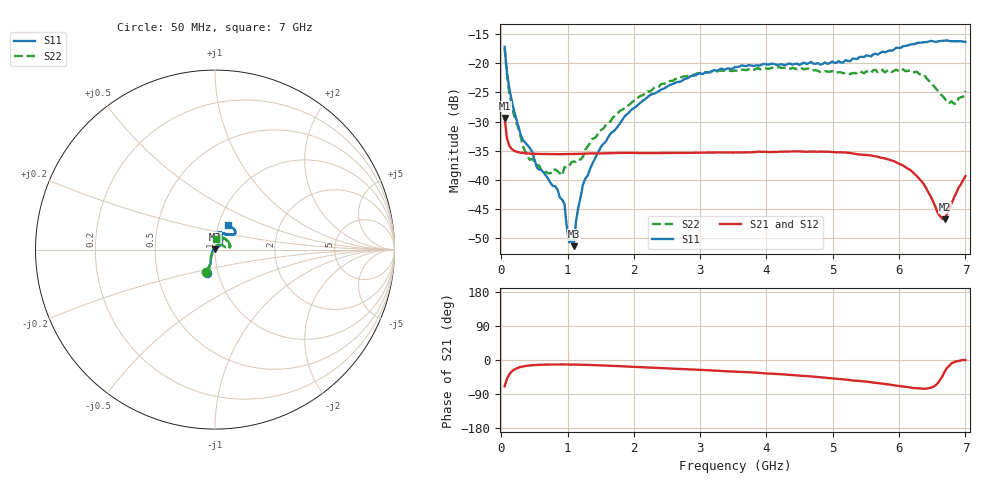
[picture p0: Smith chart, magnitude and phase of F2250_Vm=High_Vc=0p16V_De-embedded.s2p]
! Integrated Device Technology
! Corporate Headquarters
! 6024 Silver Creek Valley Road
! San Jose, CA 95138  USA
! Phone:  1-408-284-8200
! Toll Free:  1-800-223-1366
! Webpage:  http://www.idt.com/
! Timing and RF Division
! 515 Groton Road, Suite 102
! Westford, MA 01886-6024
! Device:  F2250
! Description: Voltage Variable RF Attenuator
! Frequency:  50.0 -  6000.00 MHz
! Package:  3x3 mm Thin QFN Plastic Package: 16 pin
! Ports:  2 RF, 3 DC
!  Pin  1  = GND
!  Pin  2  = NC
!  Pin  3  = RF1  = Port 1
!  Pin  4  = NC
!  Pin  5  = GND
!  Pin  6  = GND
!  Pin  7  = GND
!  Pin  8  = GND
!  Pin  9  = NC
!  Pin 10  = RF2  = Port 2
!  Pin 11  = NC
!  Pin 12  = GND
!  Pin 13  = GND
!  Pin 14  = VCNTRL
!  Pin 15  = VDD
!  Pin 16  = VMODE
! Vcntrl:  0.160 Volts
! Vmode:  +3.300 Volts
! Vdd:  +3.30  Volts
! Current:  1.243 mA
! Data:  The device was measured on a the F2250 evaluation board which has
!  individual transmission lines to the RF pins.  Data was collected
!  using a calibrated network analyzer.  The evaluation board was
!  de-embedded using a TRL calibration technique.
!  The reference plane is the edge of the package pin.
! Misc:  SN 10
!  Action Tracker AT0258
! Date Measured:  2014-11-26
! Date:  2015-10-15  MJV
! Note:
!  Integrated Device Technology supplies this data as a sample of measured
!  data at the package pin for this product.  Your particular data for this
!  product may vary.
!  Data was taken at 25 degrees C.
!  Integrated Device Technology reserves the right to change this data at anytime.
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# GHz S dB R 50
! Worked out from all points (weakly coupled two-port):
!   201 points, 50 MHz to 7 GHz, reference 50 ohm
!   highest |S21| = -29.38 dB at 50 MHz (marker M1); lowest = -46.8 dB at 6.687 GHz (marker M2)
!   lowest |S11| = -51.4 dB at 1.093 GHz (marker M3), VSWR 1.01, Z = 50 + j0.27 ohm
!   |S11| at or under -10 dB: start of sweep to end of sweep
!   |S22| runs from -39.2 to -17.4 dB; largest |S21 - S12| = 6.1e-05
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0.05  -17.18 -108.5  -29.38 -69.5  -29.38 -69.5  -17.37 -110.6
0.08475  -21.47 -107.4  -32.86 -50.1  -32.86 -50.1  -21.87 -109.0
0.15425  -26.23 -116.5  -34.68 -31.0  -34.68 -31.0  -27.10 -120.7
0.29325  -32.28 -127.5  -35.35 -18.4  -35.35 -18.5  -32.67 -133.5
0.3975  -34.11 -142.1  -35.48 -15.0  -35.48 -15.0  -36.08 -158.3
0.5365  -37.88 -154.8  -35.55 -12.9  -35.55 -12.9  -37.47 -179.9
0.64075  -38.79 -162.6  -35.58 -12.2  -35.58 -12.2  -38.89 160.8
0.91875  -43.41 156.0  -35.60 -11.8  -35.60 -11.8  -39.24 127.8
0.9535  -44.20 171.1  -35.60 -11.8  -35.60 -11.8  -37.83 124.2
1.023  -50.72 140.2  -35.59 -11.9  -35.59 -11.9  -37.71 108.2
1.0925  -51.38 88.7  -35.57 -12.0  -35.57 -12.0  -36.87 98.6
1.12725  -47.10 62.0  -35.56 -12.1  -35.56 -12.1  -36.90 91.7
1.2315  -40.84 41.0  -35.52 -12.5  -35.52 -12.5  -36.05 77.3
1.6485  -32.03 41.2  -35.44 -15.2  -35.43 -15.2  -29.92 60.0
2.37825  -24.76 46.7  -35.39 -21.0  -35.40 -21.1  -24.02 53.9
3.525  -20.66 71.7  -35.32 -30.6  -35.32 -30.6  -21.26 73.0
4.7065  -20.06 72.0  -35.16 -43.9  -35.15 -43.9  -21.21 70.4
5.85325  -17.79 40.5  -36.58 -64.9  -36.58 -64.9  -21.13 23.4
6.305  -16.47 40.4  -39.82 -75.3  -39.83 -75.3  -21.87 8.5
6.68725  -16.11 47.9  -46.80 -31.0  -46.77 -30.7  -26.03 28.4
6.861  -16.22 54.5  -42.32 -3.7  -42.27 -3.7  -26.96 57.4
7  -16.32 62.4  -39.35 -0.1  -39.33 -0.3  -24.82 83.6
